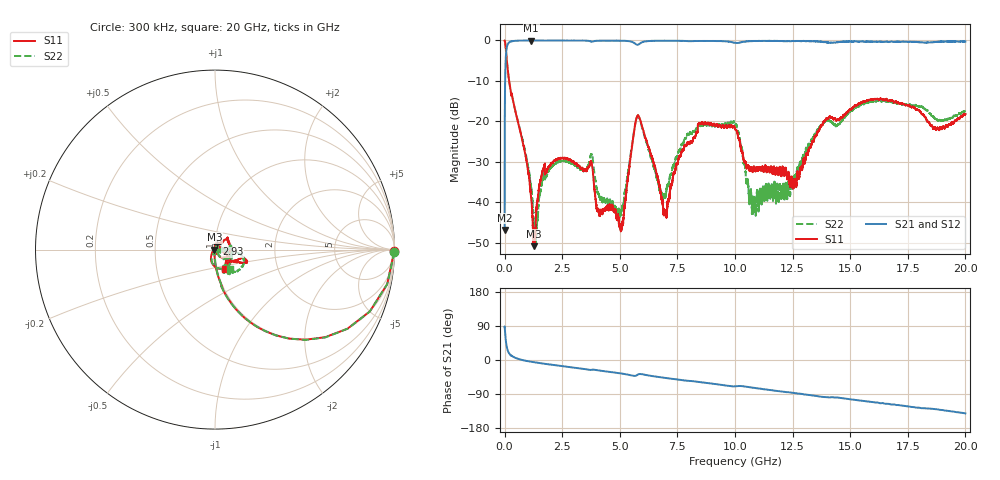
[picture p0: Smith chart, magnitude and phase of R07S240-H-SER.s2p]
!{R07S240}
!Johanson Technology Inc.
!www.johansontechnology.com
!Test Board Conditions:
!Substrate Type  RO4350B
!Substrate Thickness  10 mil
!Substrate Dk  3.66
!TL Type: GCPW
!TL Trace Width  21 mil
!TL Gap  20 mil
!Electrode orientation  Horizontal
!DUT TOPOLOGY	SERIES
!Mounting Pad LxW  16x21 mil
! Created Sat Feb  6 11:51:57 2021
# hz S ma R 50
! 2 Port Network Data from SP1.SP block
! freq  magS11  angS11  magS21  angS21  magS12  angS12  magS22  angS22
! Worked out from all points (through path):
!   20001 points, 300 kHz to 20 GHz, reference 50 ohm
!   highest |S21| = -0.01 dB at 1.154 GHz (marker M1); lowest = -46.8 dB at 300 kHz (marker M2)
!   group delay of S21, straight-line fit = 20.2 ps
!   lowest |S11| = -50.8 dB at 1.283 GHz (marker M3), VSWR 1.01, Z = 49.7 + j0.0359 ohm
!   |S11| at or under -10 dB: 195.3 MHz to end of sweep
!   |S22| runs from -49.9 to 0.0 dB; largest |S21 - S12| = 0.012
!   S11 on the Smith chart (normalised r, x): 300 kHz: open; 2.93 GHz: 1.02, +0.06; 20 GHz: 1.10, -0.24
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300000  0.9978 -0.6  0.004573 88.4  0.004539 88.9  1 -0.8
1.013e8  0.5449 -57.6  0.8345 32.8  0.8355 32.7  0.5466 -57.5
1.453e8  0.412 -66.8  0.9084 23.7  0.9085 23.7  0.411 -66.7
1.1543e9  0.01119 -107.4  0.9987 -4.6  0.9963 -4.7  0.01513 -87.1
1.2833e9  0.002876 172.8  0.9981 -5.9  0.9973 -5.9  0.00481 -70.1
1.6493e9  0.02457 91.0  0.997 -9.3  0.9966 -9.2  0.01901 65.8
2.9303e9  0.03204 73.9  0.996 -19.5  0.9972 -19.5  0.02982 57.4
3.3343e9  0.02634 70.1  0.9953 -22.7  0.9964 -22.6  0.02554 47.9
3.7693e9  0.03098 2.4  0.9667 -26.0  0.9671 -26.0  0.03947 -1.6
4.0633e9  0.008044 -108.8  0.9916 -27.3  0.9914 -27.3  0.01283 -64.4
5.0603e9  0.004448 -59.7  0.9905 -35.7  0.9908 -35.6  0.007662 -36.3
5.7963e9  0.1179 -59.0  0.886 -38.2  0.8861 -38.2  0.1178 -59.1
6.6673e9  0.01905 -138.3  0.991 -44.7  0.9921 -44.7  0.01799 -100.9
6.9763e9  0.007965 149.9  0.9927 -47.3  0.993 -47.3  0.01181 -35.6
8.4873e9  0.09378 43.9  0.9844 -58.4  0.9851 -58.4  0.08835 15.3
1.00003e10  0.08231 -17.7  0.9335 -69.6  0.9347 -69.6  0.09194 -25.7
1.08233e10  0.02655 -53.8  0.9845 -73.4  0.987 -73.5  0.009763 11.6
1.25813e10  0.01882 -43.4  0.9798 -87.0  0.9816 -87.1  0.02101 -6.2
1.33343e10  0.05335 -18.9  0.9778 -93.3  0.9795 -93.4  0.0605 -8.8
1.66673e10  0.1789 -19.6  0.9547 -115.8  0.961 -116.2  0.1778 -39.2
1.87883e10  0.08375 -35.6  0.9604 -130.2  0.9607 -130.4  0.1035 -62.9
2e10  0.1231 -61.7  0.9701 -140.8  0.9632 -140.8  0.1358 -51.5
